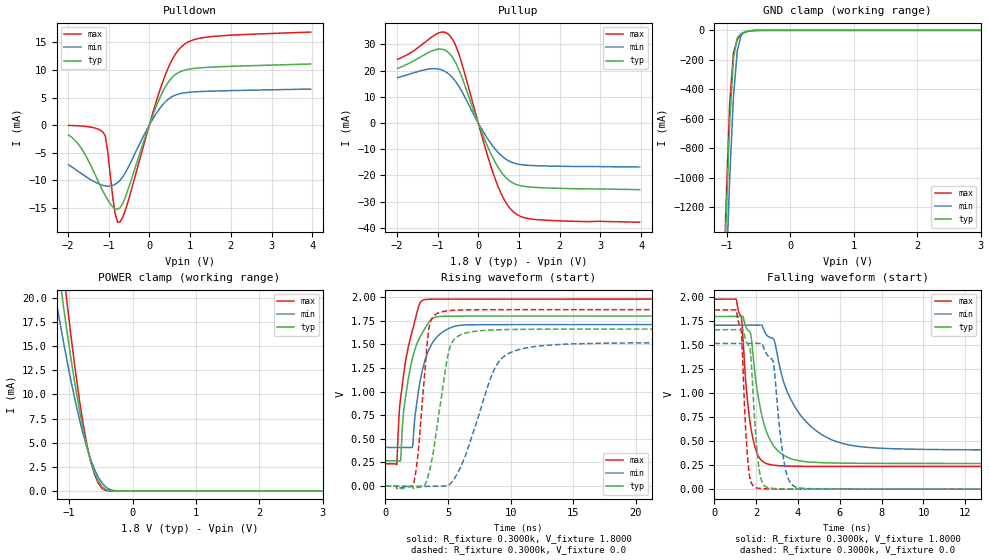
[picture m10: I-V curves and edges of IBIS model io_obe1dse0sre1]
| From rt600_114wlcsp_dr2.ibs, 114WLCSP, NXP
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[Model] io_obe1dse0sre1
|   Model io_obe1dse0sre1
| Library cells for typ/min/max conditions are connected as defined below:
|  pad - External Pad
|  ipp_do - Core Input
|  ipp_obe - Output Buffer Enable
|  REFH3V3 - vdd1v8
|  REFL3V3 - REFL3V3
|  gnde - gnde
|  ipp_ina235_3v - NC
|  ipp_ina40_3v - NC
|  ipp_ina_mux - NC
|  ipp_ind - NC
|  ipp_ind_1p8v - NC
|  ipp_ind_3v - NC
|  ipp_sre - vdd
|  vdd - vdd
|  vdd1v8 - vdd1v8
|  vdda - vdde3v3
|  vdde3v3 - vdde3v3
| All other pins connected to ground
Model_type I/O
Polarity   Non-Inverting
Enable   Active-High
Vinl =   0.5400V
Vinh =   1.2600V
Vmeas =  0.9000V
Cref =   25.0000pF
Rref =   0.5000k
Vref =   0.0V
C_comp   2.2457pF   2.1702pF   2.3896pF
[Temperature Range]   25.0000   0.1250k   -40.0000
[Voltage Range]   1.8000V   1.7100V   1.9800V
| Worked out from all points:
|   slope of the pulldown table from 0 to 0.27 V, typ, clamps not added: 52.6 ohm
|   slope of the pullup table from 0 to 0.27 V, typ, clamps not added: 26.1 ohm
|   GND clamp passes 1 mA (typ) near -0.57 V on its own axis
|   POWER clamp passes 1 mA (typ) near -0.54 V on its own axis
|   rising waveform, R_fixture 0.3000k, V_fixture 1.8000: 20-80 % time 1.15ns typ, 1.18ns min, 1.1ns max; typ from 0.268 V to 1.8 V
|   rising waveform, R_fixture 0.3000k, V_fixture 0.0: 20-80 % time 1.13ns typ, 2.3ns min, 696ps max; typ from 0 V to 1.66 V
|   falling waveform, R_fixture 0.3000k, V_fixture 1.8000: 20-80 % time 732ps typ, 1.58ns min, 438ps max; typ from 1.8 V to 0.268 V
|   falling waveform, R_fixture 0.3000k, V_fixture 0.0: 20-80 % time 309ps typ, 438ps min, 244ps max; typ from 1.66 V to 0 V
[Pulldown]
|Voltage   I(typ)   I(min)   I(max)
-1.98V    -1.78mA    -7.2mA     -50uA
-1.62V    -4.76mA    -9.02mA    -180uA
-1.08V    -12.8mA    -11.03mA   -1.913mA
-840mV    -15.17mA   -10.75mA   -15.99mA
-780mV    -15.26mA   -10.45mA   -17.61mA
-720mV    -15.01mA   -10.02mA   -17.56mA
-540mV    -12.09mA   -7.995mA   -14.33mA
240mV     4.642mA    2.876mA    5.906mA
540mV     8.479mA    5.085mA    11.58mA
780mV     9.757mA    5.756mA    14.15mA
1.44V     10.49mA    6.149mA    16mA
3.96V     11.09mA    6.548mA    16.88mA
[Pullup]
|Voltage   I(typ)   I(min)   I(max)
-1.98V    20.86mA    17.3mA     24.34mA
-1.02V    28.11mA    20.69mA    34.03mA
-840mV    27.98mA    19.9mA     34.7mA
-660mV    25.66mA    17.79mA    32.62mA
-540mV    22.59mA    15.51mA    29.07mA
-420mV    18.25mA    12.55mA    23.63mA
60mV      -2.453mA   -1.657mA   -3.359mA
420mV     -15.1mA    -10.03mA   -21.54mA
660mV     -20.53mA   -13.6mA    -29.86mA
960mV     -23.61mA   -15.64mA   -35.03mA
1.62V     -24.74mA   -16.38mA   -37.06mA
3.96V     -25.43mA   -16.79mA   -37.85mA
[GND_clamp]
|Voltage   I(typ)   I(min)   I(max)
-1.98V    -17.57A    -17.55A    -18.13A
-1.08V    -2.185A    -2.567A    -2.121A
-1.02V    -1.339A    -1.74A     -1.223A
-960mV    -630.1mA   -1.012A    -499.4mA
-900mV    -189.5mA   -452.2mA   -152mA
-840mV    -51.34mA   -139.9mA   -62.86mA
-780mV    -22.28mA   -35.54mA   -26.58mA
-720mV    -10.62mA   -11.15mA   -13.18mA
-600mV    -1.527mA   -2.152mA   -2.249mA
-480mV    -85.63uA   -243.9uA   -63.17uA
3.96V     0A         0A         0A
[POWER_clamp]
|Voltage   I(typ)   I(min)   I(max)
-1.98V    66.18mA    51.42mA    77.85mA
-1.26V    27.66mA    21.8mA     33.09mA
-1.2V     24.56mA    19.48mA    29.34mA
-1.14V    21.54mA    17.24mA    25.67mA
-1.08V    18.63mA    15.07mA    22.11mA
-1.02V    15.84mA    13mA       18.69mA
-840mV    8.434mA    7.464mA    9.5mA
-720mV    4.556mA    4.476mA    4.785mA
-600mV    1.876mA    2.218mA    1.703mA
-540mV    1.008mA    1.402mA    786.9uA
-420mV    135uA      383.7uA    43.39uA
3.96V     0A         0A         0A
[Ramp]
| variable   typ   min   max
dV/dt_r  0.6454/2.4919n   0.4663/4.9402n   0.8344/1.3801n
dV/dt_f  0.3124/1.8985n   0.1842/2.5269n   0.4711/1.0697n
R_load = 50.0000
[Rising Waveform]
R_fixture= 0.3000k
V_fixture= 1.8000
V_fixture_min= 1.7100
V_fixture_max= 1.9800
|time   V(typ)   V(min)   V(max)
0s        267.9mV    408.9mV    235.9mV
898.3ps   267.9mV    408.9mV    227.2mV
1.201ns   266.6mV    408.9mV    918.2mV
1.452ns   797.9mV    408.9mV    1.186V
2.15ns    1.349V     410mV      1.645V
2.726ns   1.569V     1.079V     1.929V
3.536ns   1.746V     1.464V     1.978V
5.099ns   1.799V     1.671V     1.98V
7.939ns   1.8V       1.709V     1.98V
500ns     1.8V       1.71V      1.98V
[Rising Waveform]
R_fixture= 0.3000k
V_fixture= 0.0
V_fixture_min= 0.0
V_fixture_max= 0.0
|time   V(typ)   V(min)   V(max)
0s        65.02nV    1.918uV    111.1nV
2.223ns   -4.78mV    -23.18mV   17.11mV
2.623ns   -2.104mV   -13.14mV   368.4mV
3.198ns   23.29mV    -4.817mV   1.301V
3.757ns   311.6mV    -1.86mV    1.785V
5.03ns    1.406V     7.679mV    1.857V
6.001ns   1.601V     199mV      1.864V
9.427ns   1.656V     1.368V     1.868V
16.14ns   1.662V     1.509V     1.868V
500ns     1.662V     1.519V     1.868V
[Falling Waveform]
R_fixture= 0.3000k
V_fixture= 1.8000
V_fixture_min= 1.7100
V_fixture_max= 1.9800
|time   V(typ)   V(min)   V(max)
0s        1.8V       1.71V      1.98V
1.032ns   1.8V       1.71V      1.981V
1.275ns   1.799V     1.71V      1.802V
1.649ns   1.648V     1.71V      786mV
2.075ns   988mV      1.709V     355.8mV
2.758ns   474.7mV    1.575V     252.3mV
3.954ns   299.7mV    821.5mV    238.2mV
6.367ns   270.5mV    464mV      236.1mV
12.53ns   268mV      410.3mV    236mV
500ns     267.9mV    408.9mV    235.9mV
[Falling Waveform]
R_fixture= 0.3000k
V_fixture= 0.0
V_fixture_min= 0.0
V_fixture_max= 0.0
|time   V(typ)   V(min)   V(max)
0s        1.662V     1.519V     1.868V
1.266ns   1.661V     1.519V     1.68V
1.509ns   1.546V     1.519V     562.4mV
1.685ns   1.484V     1.519V     132.9mV
2.154ns   183.7mV    1.519V     7.536mV
2.801ns   7.617mV    1.335V     2.039mV
3.195ns   4.131mV    484.7mV    1.047mV
3.518ns   2.934mV    116.8mV    639.9uV
5.265ns   602uV      3.351mV    70.91uV
500ns     1.128uV    3.18uV     781.6nV
